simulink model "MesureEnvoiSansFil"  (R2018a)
settings: Solver=ode45  StartTime=0.0  StopTime=10.0  RelTol=1e-3  EnableMultiTasking=on
libraries: arduinolib x2, arduinowifilib x1

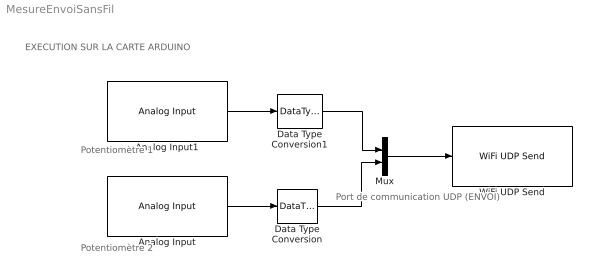
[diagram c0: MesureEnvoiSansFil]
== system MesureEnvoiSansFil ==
  note: Potentiomètre 1
  note: Potentiomètre 2
  note: Port de communication UDP (ENVOI)
  note: EXECUTION SUR LA CARTE ARDUINO
  Analog Input : arduinolib/Analog Input  pinNumber=1  ReadResultsOnly=off  ConversionTriggerSource=Software  ExternalTriggerType=uint32(0)  OutputDataType=uint16  EnableConversionCompleteNotify=off  EnableOuputStatus=off  SampleTime=0.01  blockPlatform=arduino
  Analog Input1 : arduinolib/Analog Input  pinNumber=0  ReadResultsOnly=off  ConversionTriggerSource=Software  ExternalTriggerType=uint32(0)  OutputDataType=uint16  EnableConversionCompleteNotify=off  EnableOuputStatus=off  SampleTime=0.01  blockPlatform=arduino
  Data Type Conversion : DataTypeConversion  OutDataTypeStr=uint16
  Data Type Conversion1 : DataTypeConversion  OutDataTypeStr=uint16
  Mux : Mux  Inputs=2
  WiFi UDP Send : arduinowifilib/WiFi UDP Send  remoteIPOctetString=192.168.1.33  remoteport=50002  localport=50001  remoteipoctet1=192  remoteipoctet2=168  remoteipoctet3=1  remoteipoctet4=33  wifiUDPIndex=0  blockPlatform=arduino  isARMArch=false
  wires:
  Data Type Conversion/1 -> Mux/2
  Mux/1 -> WiFi UDP Send/1
  Analog Input/1 -> Data Type Conversion/1
  Analog Input1/1 -> Data Type Conversion1/1
  Data Type Conversion1/1 -> Mux/1
